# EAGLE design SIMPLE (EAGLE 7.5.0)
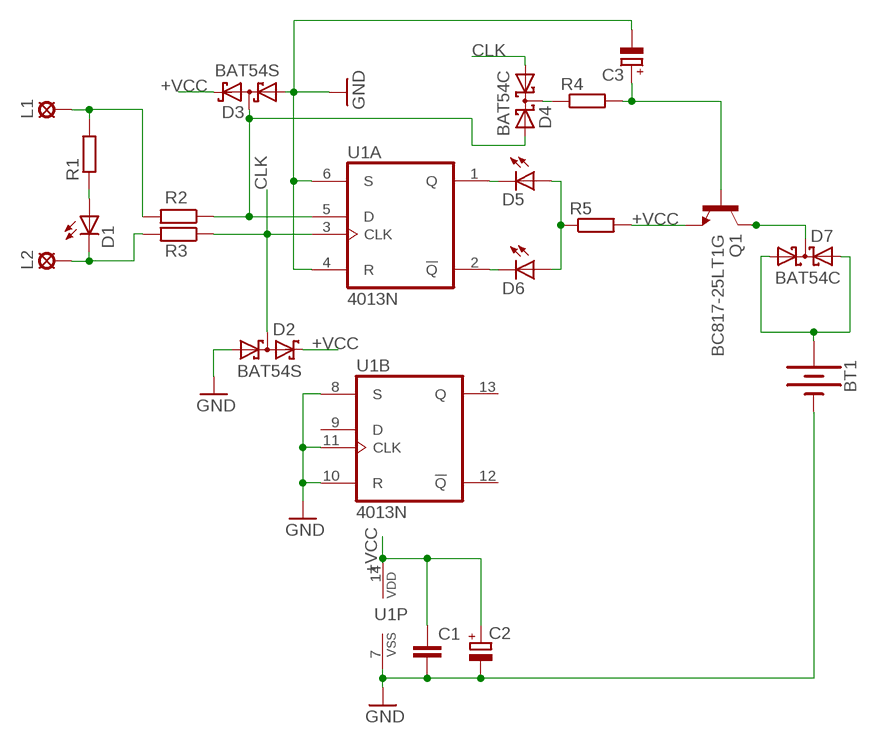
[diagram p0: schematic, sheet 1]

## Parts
BT1  BATTERY-9V  [BATTCON_9V]
C1  C-EUC1206  [C1206]
C2  CPOL-EUSMCC  [SMC_C]
C3  CPOL-EUSMCC  [SMC_C]
D1  LED5MM  [LED5MM]
D2  BAT54S  [SOT23]
D3  BAT54S  [SOT23]
D4  BAT54C  [SOT23]
D5  LED5MM  [LED5MM]
D6  LED5MM  [LED5MM]
D7  BAT54C  [SOT23]
L1  LSP13  [LSP13]
L2  LSP13  [LSP13]
Q1  BC817-25LT1G  [SOT95P237X111-3N]
R1  R-EU_R2512  [R2512]
R2  R-EU_R2512  [R2512]
R3  R-EU_R2512  [R2512]
R4  R-EU_M1206  [M1206]
R5  R-EU_M1206  [M1206]
U1  4013N  [DIL14]

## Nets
+VCC: C1.1 C2.+ D2.2(C2) D3.2(C2) Q1.2(E) R5.2 U1.14(P:VDD)
CLK: D2.3(C1A2) D4.1(A1) R3.1 U1.3(A:CLK)
GND: BT1.- C1.2 C2.- C3.- D2.1(A1) D3.1(A1) U1.4(A:R) U1.6(A:S) U1.7(P:VSS) U1.8(B:S) U1.10(B:R) U1.11(B:CLK)
N$1: L1.MP R1.2 R2.2
N$2: D1.A R1.1
N$3: D1.K(C) L2.MP R3.2
N$4: D3.3(C1A2) D4.2(A2) R2.1 U1.5(A:D)
N$5: D4.3(CC) R4.1
N$6: D5.K(C) U1.1(A:Q)
N$7: D6.K(C) U1.2(A:!Q)
N$8: D5.A D6.A R5.1
N$9: C3.+ Q1.1(B) R4.2
N$11: D7.3(CC) Q1.3(C)
N$24: BT1.+ D7.1(A1) D7.2(A2)
Unconnected: U1.9(B:D) U1.12(B:!Q) U1.13(B:Q)

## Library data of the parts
BT1 = SparkFun-Batteries:BATTERY: Battery - Single Cell; PROD_ID: BATT-10855
C1 = rcl:C-EU: CAPACITOR, European symbol
C2 C3 = rcl:CPOL-EU: POLARIZED CAPACITOR, European symbol
D1 D5 D6 = led:LED: LED
D2 D3 = diode:BAT54S: Schottky Diodes Pin connection corrected 2011-05-04 Source: Fairchild .. BAT54.pdf
D4 D7 = diode:BAT54C: Schottky Diodes Source: Fairchild .. BAT54.pdf
L1 L2 = solpad:LSP13: SOLDER PAD
Q1 = BC817-25LT1G:BC817-25LT1G: Check availability; AVAILABILITY: In Stock; CHECK_PRICES: https://www.snapeda.com/parts/BC817-25LT1G/Onsemi/view-part/?ref=eda; DESCRIPTION: Transistor NPN 45V 0.5A hfe160 SOT23 | ON Semiconductor BC817-25LT1G; MF: ON Semiconductor; MP: BC817-25LT1G; PACKAGE: SOT-23-3 ON Semiconductor; PRICE: None; PURCHASE-URL: https://www.snapeda.com/api/url_track_click_mouser/?unipart_id=343725&manufacturer=ON Semiconductor&part_name=BC817-25LT1G&search_term=transistor sot23; SNAPEDA_LINK: https://www.snapeda.com/parts/BC817-25LT1G/Onsemi/view-part/?ref=snap
R1-R5 = rcl:R-EU_: RESISTOR, European symbol
U1 = 40xx:4013: Dual D FLIP FLOP, set/reset

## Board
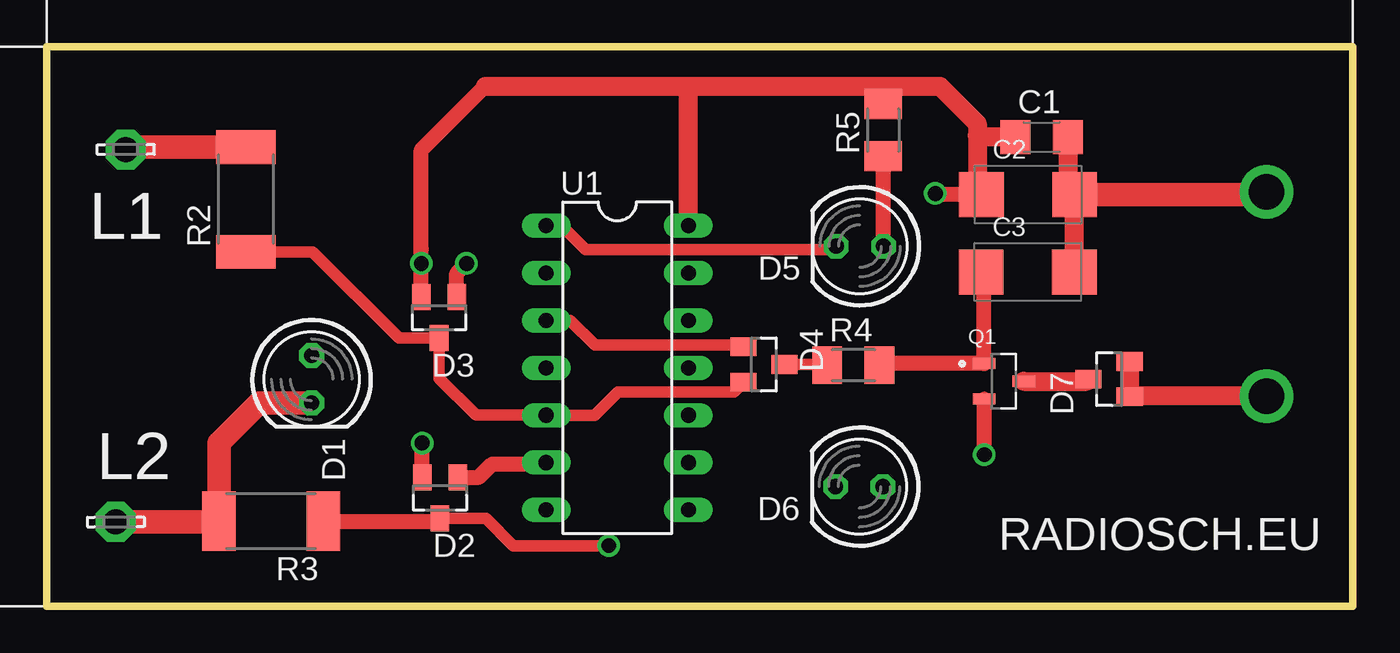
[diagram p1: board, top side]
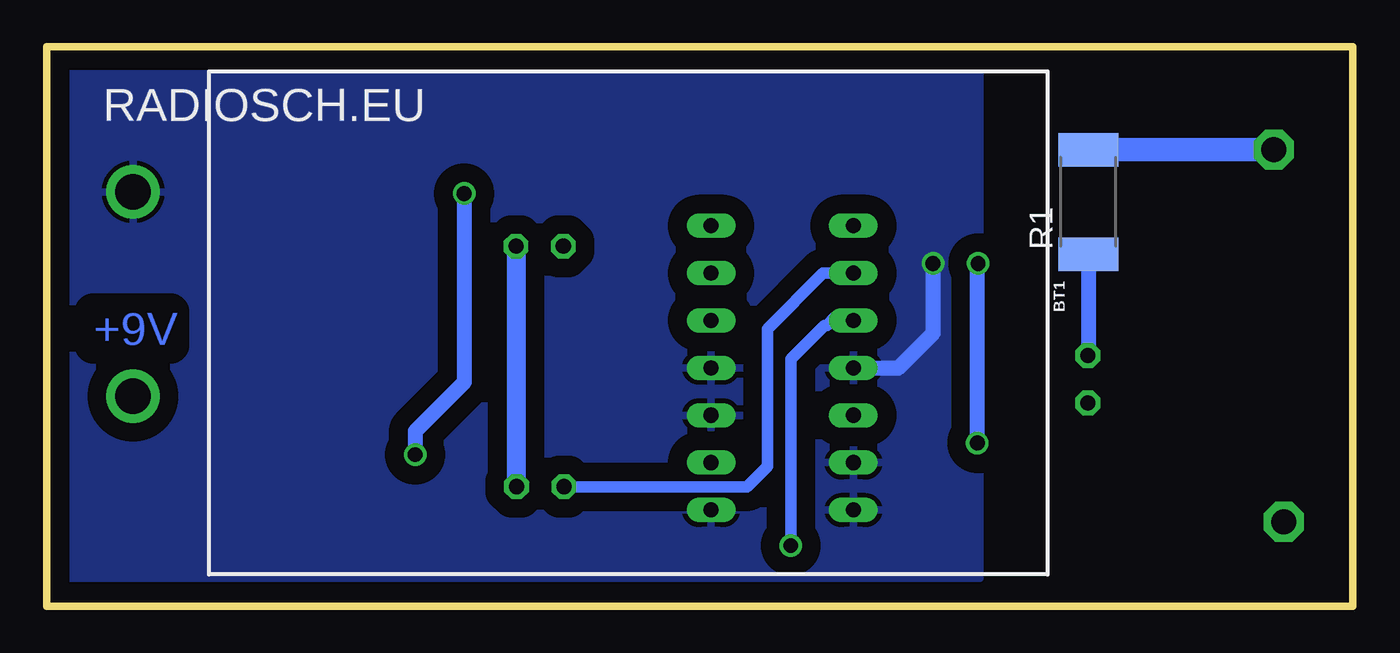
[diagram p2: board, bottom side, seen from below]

Size 70 x 30 mm. Coordinates in mm from the lower left corner, seen from the top.
Outline: 0,0 70,0 70,30 0,30 0,0
Copper layers (1*16): Top 0.035mm / dielectric 1.5mm / Bottom 0.035mm
Design rules "default": minimum track width 10mil, minimum drill 24mil, track to track 8mil, track to pad 8mil, pad to pad 8mil, via to via 8mil, smd to smd 8mil, copper to edge 40mil, drill to drill 8mil, minimum pad ring 10mil, minimum via ring 8mil, stop-mask expansion 4mil, vias tented up to drill 0mil, thermal gap 10mil

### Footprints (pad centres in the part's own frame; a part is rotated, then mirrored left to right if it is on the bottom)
BATTCON_9V = drill 1.905: + -4,-1; - -4,-11.954
C1206 = smd 1.6 x 1.8: 1 -1.4,0; 2 1.4,0
SMC_C = smd 2.4 x 2.4: + -2.5,0; - 2.5,0
LED5MM = drill 0.813 octagon: A -1.27,0; K 1.27,0
SOT23 = smd 1 x 1.4: 1 -0.95,-1.1; 2 0.95,-1.1; 3 0,1.1
LSP13 = drill 1.321 pad 2.159 octagon: MP 0,0
SOT95P237X111-3N = smd 1.23 x 0.6: 1 -1.06,0.95; 2 -1.06,-0.95; 3 1.06,0
R2512 = smd 1.8 x 3.2: 1 -2.8,0; 2 2.8,0
M1206 = smd 1.6 x 2: 1 -1.4,0; 2 1.4,0
DIL14 = drill 0.813 long: 1 -7.62,-3.81; 2 -5.08,-3.81; 3 -2.54,-3.81; 4 0,-3.81; 5 2.54,-3.81; 6 5.08,-3.81; 7 7.62,-3.81; 8 7.62,3.81; 9 5.08,3.81; 10 2.54,3.81; 11 0,3.81; 12 -2.54,3.81; 13 -5.08,3.81; 14 -7.62,3.81

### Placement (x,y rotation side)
BT1  69.37,10.26 180 bottom
C1  53.32,25.15 0 top
C2  52.59,22.07 0 top
C3  52.58,17.92 0 top
D1  14.2,12.17 270 top
D2  21.08,5.81 180 top
D3  21.03,15.47 180 top
D4  38.44,12.96 270 top
D5  43.58,19.3 180 top
D6  43.55,6.41 180 top
D7  56.94,12.18 90 top
L1  4.24,24.48 180 top
L2  3.7,4.52 0 top
Q1  51.3,12.06 0 top
R1  14.18,21.67 90 bottom
R2  10.68,21.81 90 top
R3  12.03,4.56 180 top
R4  43.23,12.92 0 top
R5  44.83,25.52 90 top
U1  30.58,12.78 270 top

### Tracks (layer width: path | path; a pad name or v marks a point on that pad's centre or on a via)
+VCC  (via drill 0.8)
  Top 0.813: D3.2 v20.08,18.38 20.08,19.12 20.08,24.45 23.5,27.88 | C2.+ 47.68,22.07 v47.62,22.12 | v50.25,8.12 Q1.2 | D2.2 v20.13,8.75 v20.12,8.75
  Top 1.016: 23.5,27.88 34.62,27.88 | 34.62,27.88 45,27.88 | 45,27.88 47.88,27.88 49.88,25.88 49.88,25.25 | 49.88,25.25 49.88,22.29 C2.+ | U1.14 34.39,27.64 34.62,27.88 | R5.2 44.83,27.7 45,27.88 | C1.1 49.98,25.15 49.88,25.25
  Bottom 0.813: v47.62,22.12 47.62,12 50.25,9.38 v50.25,8.12 | v20.12,8.75 20.12,18.33 v20.08,18.38
CLK  (via drill 0.8)
  Top 0.61: U1.3 28.05,15.32 29.38,14 37.24,14 D4.1 | D2.3 23.54,4.71 25,3.25 v30.12,3.25
  Top 0.813: R3.1 20.93,4.56 D2.3
  Bottom 0.61: v30.12,3.25 30.12,13.25 28.31,15.06 28.19,15.06 27.75,15.5 26.95,15.5 U1.3
GND  (via drill 0.8)
  Top 0.813: D3.1 21.98,17.86 v22.5,18.38 | D2.1 23.16,6.91 23.88,7.62 26.7,7.62 U1.6
  Top 1.016: C1.2 54.72,22.44 C2.- C3.-
  Top 1.27: C2.- 65.23,22.07 BT1.-
  Bottom 0.813: v22.5,18.38 22.5,14.62 24.38,12.75 26.74,12.75 U1.4
  pour Bottom (isolate 1): 20,29 70,29 70,1.5 20,1.5
N$1
  Top 1.27: R2.2 4.37,24.61 L1.MP
  Bottom 1.27: R1.2 L1.MP
N$2
  Bottom 0.813: R1.1 14.18,13.46 D1.A
N$3
  Top 1.27: L2.MP 9.19,4.52 R3.2 9.25,4.58 9.25,8.75 11.4,10.9 D1.K
N$4
  Top 0.61: R2.1 14.25,19 18.88,14.37 D3.3 21.03,12.22 23,10.25 U1.5 29.36,10.24 30.62,11.5 36.83,11.5 D4.2
N$5
  Top 0.61: D4.3 41.79,12.96 R4.1
N$6
  Top 0.61: U1.1 27.6,20.4 28.88,19.12 42.13,19.12 D5.K
N$7
  Bottom 0.61: D6.K 32.47,6.41 31.38,7.5 31.38,14.88 28.39,17.86 U1.2
N$8
  Top 0.813: D5.A 44.85,24.11 R5.1
  Bottom 1.016: D5.A 44.85,6.44 D6.A
N$9
  Top 0.813: R4.2 44.72,13.01 Q1.1 50.24,17.76 C3.+
N$11
  Top 1.016: Q1.3 55.72,12.06 D7.3
N$24
  Top 1.016: D7.2 D7.1 58.07,11.26 BT1.+

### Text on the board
Bottom: +9V
tPlace: RADIOSCH.EU
bPlace: RADIOSCH.EU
